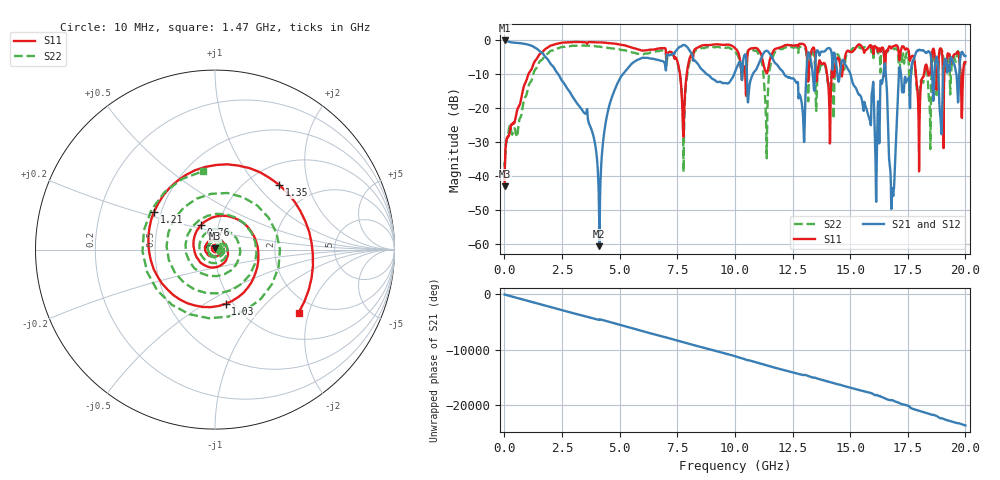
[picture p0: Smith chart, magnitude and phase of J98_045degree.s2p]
!Keysight Technologies,N5222A,MY51421036,A.10.65.16
!Date: Friday, March 31, 2023 15:15:50
!Correction: S11(Full 2 Port(1,2))
!S21(Full 2 Port(1,2))
!S12(Full 2 Port(1,2))
!S22(Full 2 Port(1,2))
!S2P File: Measurements: S11, S21, S12, S22:
# Hz S  dB  R 50
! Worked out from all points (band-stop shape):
!   2000 points, 10 MHz to 20 GHz, reference 50 ohm
!   highest |S21| = -0.03 dB at 10 MHz (marker M1); lowest = -60.5 dB at 4.12 GHz (marker M2)
!   |S21| within 3 dB of the highest: start of sweep to 1.501 GHz; 7.45 GHz to 8.036 GHz (585.7 MHz wide, 7.56 % of centre)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
!   lowest |S11| = -42.9 dB at 10 MHz (marker M3), VSWR 1.01, Z = 50.2 + j0.691 ohm
!   |S11| at or under -10 dB: start of sweep to 1.042 GHz; 7.621 GHz to 7.91 GHz (288.5 MHz wide, 3.71 % of centre); 17.85 GHz to 18.2 GHz (345.6 MHz wide, 1.92 % of centre)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
!   |S22| runs from -38.7 to -1.5 dB; largest |S21 - S12| = 0.012
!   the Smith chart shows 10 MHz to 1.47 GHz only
!   S11 on the Smith chart (normalised r, x): 10 MHz: 1.00, +0.01; 760 MHz: 0.83, +0.23; 1.03 GHz: 0.93, -0.62; 1.21 GHz: 0.46, +0.23; 1.35 GHz: 1.36, +1.33; 1.47 GHz: 1.61, -1.72
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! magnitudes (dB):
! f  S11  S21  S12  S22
! 10 MHz  -42.9  0.0  0.0  -35.7
! 760 MHz  -16.0  -0.9  -0.9  -21.2
! 1.03 GHz  -10.2  -1.3  -1.3  -14.0
! 1.21 GHz  -8.0  -1.7  -1.6  -11.1
! 1.35 GHz  -5.9  -2.2  -2.2  -8.4
! 1.47 GHz  -4.7  -2.8  -2.8  -7.1
! 3.35 GHz  -0.5  -20.3  -20.2  -1.6
! 4.12 GHz  -0.6  -60.5  -59.5  -1.9
! 4.91 GHz  -1.1  -12.6  -12.6  -2.6
! 6.68 GHz  -2.4  -5.8  -5.8  -3.2
! 7.77 GHz  -28.3  -1.4  -1.3  -38.7
! 10.01 GHz  -2.3  -9.2  -9.2  -3.2
! 11.36 GHz  -9.5  -3.1  -3.1  -25.8
! 13.34 GHz  -2.8  -7.9  -7.9  -4.0
! 16.17 GHz  -2.3  -29.4  -29.3  -2.8
! 16.48 GHz  -5.1  -7.6  -7.6  -5.2
! 16.67 GHz  -2.1  -31.1  -31.0  -2.8
! 16.85 GHz  -1.8  -45.0  -44.5  -2.2
! 17.14 GHz  -5.9  -7.9  -7.9  -10.2
! 17.92 GHz  -14.8  -3.0  -2.9  -15.3
! 18.93 GHz  -2.3  -23.7  -23.8  -3.5
! 20 GHz  -6.4  -4.6  -4.6  -7.2
